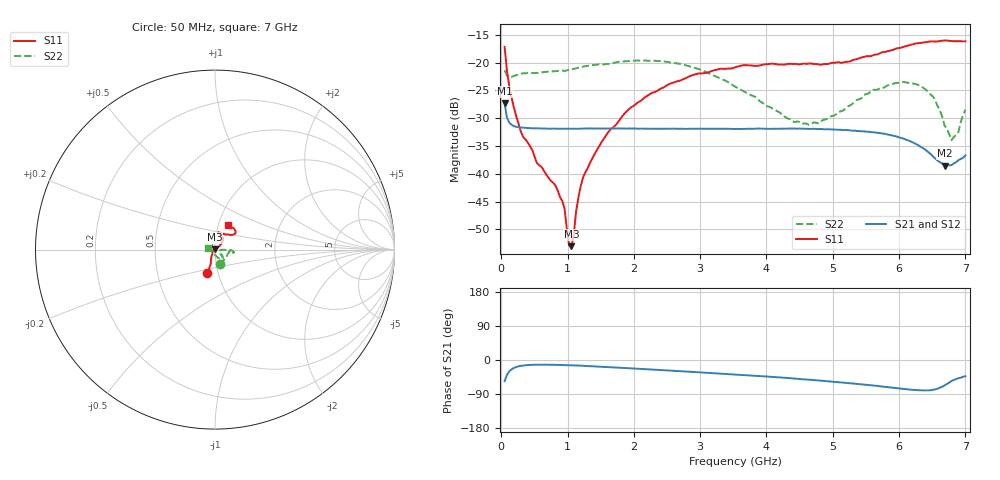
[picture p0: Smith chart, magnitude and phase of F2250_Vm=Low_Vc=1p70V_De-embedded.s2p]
! Integrated Device Technology
! Corporate Headquarters
! 6024 Silver Creek Valley Road
! San Jose, CA 95138  USA
! Phone:  1-408-284-8200
! Toll Free:  1-800-223-1366
! Webpage:  http://www.idt.com/
! Timing and RF Division
! 515 Groton Road, Suite 102
! Westford, MA 01886-6024
! Device:  F2250
! Description: Voltage Variable RF Attenuator
! Frequency:  50.0 -  6000.00 MHz
! Package:  3x3 mm Thin QFN Plastic Package: 16 pin
! Ports:  2 RF, 3 DC
!  Pin  1  = GND
!  Pin  2  = NC
!  Pin  3  = RF1  = Port 1
!  Pin  4  = NC
!  Pin  5  = GND
!  Pin  6  = GND
!  Pin  7  = GND
!  Pin  8  = GND
!  Pin  9  = NC
!  Pin 10  = RF2  = Port 2
!  Pin 11  = NC
!  Pin 12  = GND
!  Pin 13  = GND
!  Pin 14  = VCNTRL
!  Pin 15  = VDD
!  Pin 16  = VMODE
! Vcntrl:  1.700 Volts
! Vmode:  +0.000 Volts
! Vdd:  +3.30  Volts
! Current:  1.188 mA
! Data:  The device was measured on a the F2250 evaluation board which has
!  individual transmission lines to the RF pins.  Data was collected
!  using a calibrated network analyzer.  The evaluation board was
!  de-embedded using a TRL calibration technique.
!  The reference plane is the edge of the package pin.
! Misc:  SN 10
!  Action Tracker AT0258
! Date Measured:  2014-11-26
! Date:  2015-10-15  MJV
! Note:
!  Integrated Device Technology supplies this data as a sample of measured
!  data at the package pin for this product.  Your particular data for this
!  product may vary.
!  Data was taken at 25 degrees C.
!  Integrated Device Technology reserves the right to change this data at anytime.
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# GHz S dB R 50
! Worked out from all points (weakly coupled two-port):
!   201 points, 50 MHz to 7 GHz, reference 50 ohm
!   highest |S21| = -27.31 dB at 50 MHz (marker M1); lowest = -38.5 dB at 6.687 GHz (marker M2)
!   lowest |S11| = -53.0 dB at 1.058 GHz (marker M3), VSWR 1.00, Z = 49.9 + j0.211 ohm
!   |S11| at or under -10 dB: start of sweep to end of sweep
!   |S22| runs from -34.0 to -19.6 dB; largest |S21 - S12| = 0.00011
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0.05  -17.15 -108.0  -27.31 -55.9  -27.30 -55.9  -21.36 -72.2
0.1195  -24.20 -110.8  -30.78 -30.1  -30.78 -30.2  -22.52 -24.8
0.29325  -32.33 -125.6  -31.67 -15.5  -31.70 -15.6  -21.99 -11.7
0.5365  -38.05 -152.7  -31.83 -12.4  -31.84 -12.4  -21.86 -7.9
0.84925  -42.97 171.1  -31.89 -12.9  -31.90 -12.9  -21.51 -10.0
0.9535  -46.21 171.5  -31.90 -13.4  -31.90 -13.4  -21.53 -10.5
1.023  -52.93 137.7  -31.90 -13.8  -31.91 -13.8  -21.29 -10.2
1.05775  -53.03 109.0  -31.91 -14.0  -31.90 -14.0  -21.22 -10.2
1.162  -44.29 48.0  -31.89 -14.7  -31.88 -14.7  -20.92 -11.3
1.2315  -40.72 38.6  -31.86 -15.2  -31.86 -15.2  -20.72 -11.9
1.6485  -32.01 40.0  -31.85 -19.0  -31.87 -19.0  -20.20 -10.5
2.37825  -24.87 46.5  -31.91 -26.3  -31.91 -26.3  -19.71 -6.9
3.525  -20.86 72.1  -31.95 -38.2  -31.94 -38.2  -24.31 -1.8
4.39375  -20.24 76.7  -31.87 -48.6  -31.86 -48.6  -30.54 -6.7
4.7065  -20.24 72.1  -31.91 -52.9  -31.92 -52.9  -30.79 -19.6
5.85325  -17.86 40.2  -33.00 -72.1  -32.98 -72.1  -24.03 -47.0
6.3745  -16.36 41.2  -35.49 -80.2  -35.50 -80.3  -24.62 -59.1
6.5135  -16.18 44.2  -36.92 -78.7  -36.92 -78.6  -26.14 -69.6
6.68725  -16.02 48.6  -38.54 -66.8  -38.51 -66.8  -31.33 -93.5
6.7915  -16.13 52.1  -38.44 -55.2  -38.40 -55.3  -33.97 -129.5
6.89575  -16.13 56.9  -37.55 -48.0  -37.51 -48.1  -32.45 -170.1
7  -16.16 63.0  -36.70 -42.7  -36.66 -42.8  -28.48 167.7
